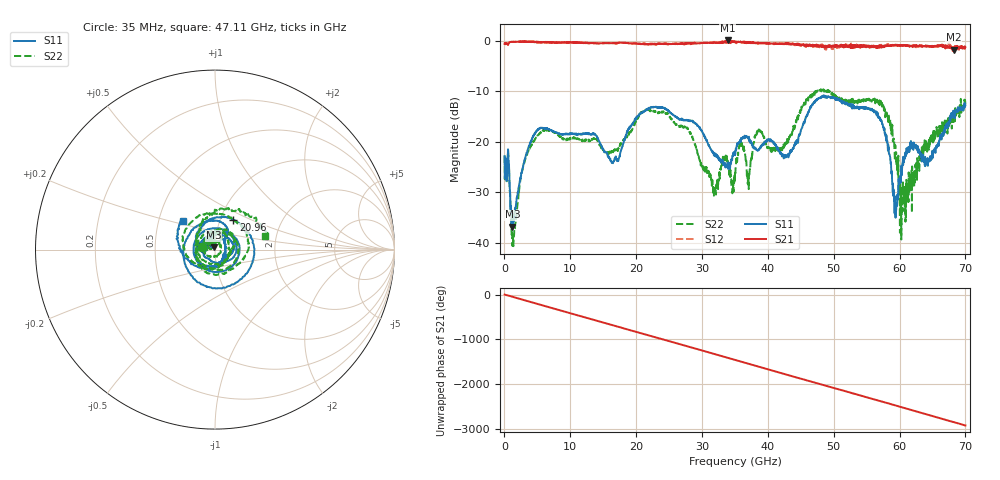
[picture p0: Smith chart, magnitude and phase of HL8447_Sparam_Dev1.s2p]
! 1/27/2023 9:40:07 AM
! D:\SMA SENSE\127\FIN\SN1.S2P
! CHANNEL.1
! TR.MEASUREMENT
! CORRECTED.DATA
# GHZ S RI R 50.0
! FREQ.GHZ  S11RE  S11IM  S21RE  S21IM  S12RE  S12IM  S22RE  S22IM
!; PortSelection: Port_12
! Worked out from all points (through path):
!   2000 points, 35 MHz to 70 GHz, reference 50 ohm
!   highest |S21| = 0.01 dB at 33.91 GHz (marker M1); lowest = -1.8 dB at 68.22 GHz (marker M2)
!   group delay of S21, straight-line fit = 116 ps
!   lowest |S11| = -36.8 dB at 1.225 GHz (marker M3), VSWR 1.03, Z = 49.3 + j1.27 ohm
!   |S11| at or under -10 dB: start of sweep to end of sweep
!   |S22| runs from -40.6 to -9.5 dB; largest |S21 - S12| = 0.1
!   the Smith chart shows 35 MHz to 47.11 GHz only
!   S11 on the Smith chart (normalised r, x): 35 MHz: 0.87, +0.03; 20.96 GHz: 1.15, +0.39; 47.11 GHz: 0.66, +0.23
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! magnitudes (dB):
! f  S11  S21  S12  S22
! 35 MHz  -22.9  -0.7  -0.7  -22.8
! 1.225 GHz  -36.8  -0.3  -0.2  -40.6
! 4.97 GHz  -17.7  -0.3  -0.3  -18.9
! 11.72 GHz  -18.5  -0.5  -0.4  -19.8
! 16.48 GHz  -24.2  -0.5  -0.5  -21.9
! 20.96 GHz  -14.3  -0.6  -0.7  -14.0
! 23.38 GHz  -13.2  -0.7  -0.6  -14.4
! 31.85 GHz  -22.2  -0.4  -0.3  -29.7
! 33.91 GHz  -24.1  0.0  -0.1  -23.5
! 35.03 GHz  -22.6  -0.3  -0.3  -25.8
! 35.88 GHz  -20.0  -0.2  -0.3  -21.0
! 37.13 GHz  -19.0  -0.3  -0.3  -26.4
! 38.5 GHz  -21.6  -0.5  -0.5  -17.9
! 42.95 GHz  -22.6  -0.5  -0.6  -19.4
! 46.69 GHz  -12.8  -1.0  -1.2  -10.6
! 47.11 GHz  -12.3  -1.0  -1.0  -10.7
! 56.1 GHz  -13.7  -1.3  -1.1  -11.6
! 58.34 GHz  -21.1  -1.1  -0.8  -14.7
! 59.4 GHz  -35.0  -0.9  -0.9  -22.4
! 60.38 GHz  -25.5  -1.0  -1.0  -28.7
! 68.22 GHz  -14.9  -1.8  -1.6  -15.3
! 70 GHz  -12.9  -1.3  -1.3  -12.7
